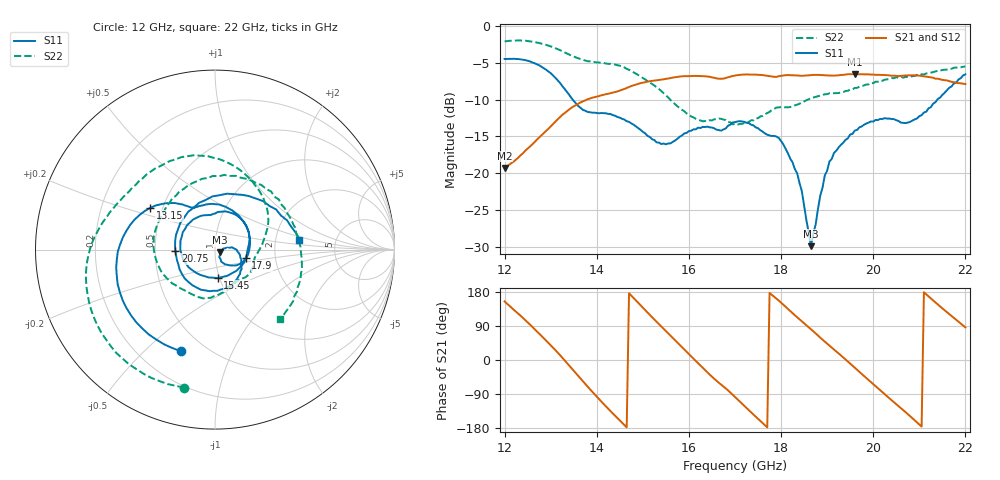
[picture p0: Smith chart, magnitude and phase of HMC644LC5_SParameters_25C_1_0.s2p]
!Analog Devices Inc..
!GaAs MMIC 5-BIT DIGITAL PHASE SHIFTER, 15 -8.5 GHz
!Filename: HMC644LC5_sparm_25C_1_0.s2p
!  :25C = 25degC
!  :_1_ = Sn1
!  :_0  = 0 state (reference)
!Device type:
!2 Port Calibration to sma connectors
!Phase Shifter:  0.000
!	TA = +25deg C, 50 Ohm System, Control Voltage = 0/-3V
!Freq	S11	S11	S21	S21	S12	S12	S22	S22
! GHz	Mag dB	Degrees	Mag dB	Degrees	Mag dB	Degrees	Mag dB	Degrees
# GHZ S DB R 50.0
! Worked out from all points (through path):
!   201 points, 12 GHz to 22 GHz, reference 50 ohm
!   highest |S21| = -6.52 dB at 19.6 GHz (marker M1); lowest = -19.3 dB at 12 GHz (marker M2)
!   lowest |S11| = -29.9 dB at 18.65 GHz (marker M3), VSWR 1.07, Z = 52.9 - j1.58 ohm
!   |S11| at or under -10 dB: 13.48 GHz to 21.39 GHz (7.912 GHz wide, 45.4 % of centre)
!   |S22| runs from -13.4 to -2.0 dB; largest |S21 - S12| = 0.0051
!   S11 on the Smith chart (normalised r, x): 12 GHz: 0.37, -0.65; 13.15 GHz: 0.43, +0.24; 15.45 GHz: 0.98, -0.32; 17.9 GHz: 1.41, -0.13; 20.75 GHz: 0.64, -0.01; 22 GHz: 2.72, +0.36
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12  -4.47 -108.7  -19.30 154.7  -19.26 154.6  -2.06 -102.5
12.55  -4.80 -160.5  -16.38 93.6  -16.39 93.7  -2.08 -140.5
13.15  -7.36 147.1  -12.70 19.9  -12.72 19.9  -3.13 -179.9
13.7  -11.40 119.5  -10.23 -56.2  -10.21 -56.2  -4.59 150.4
14.15  -11.84 97.4  -9.34 -116.2  -9.36 -116.1  -5.01 126.2
14.65  -12.93 49.6  -8.41 -177.7  -8.41 -177.5  -5.81 91.2
15.35  -15.84 -64.7  -7.32 94.5  -7.30 94.6  -8.56 39.7
15.45  -15.97 -84.2  -7.24 82.5  -7.22 82.6  -9.12 32.2
16.15  -14.03 158.3  -6.77 -2.6  -6.77 -2.5  -12.61 -5.8
16.55  -13.90 109.0  -7.03 -49.6  -7.01 -49.5  -12.67 -24.3
17  -13.06 69.7  -6.72 -97.4  -6.70 -97.3  -13.31 -52.5
17.5  -13.89 17.0  -6.62 -155.3  -6.59 -155.2  -12.52 -76.0
17.9  -15.03 -15.2  -6.90 161.8  -6.87 161.9  -11.07 -103.3
18.35  -20.02 -55.7  -6.71 112.5  -6.73 112.5  -10.67 -134.8
18.65  -29.93 -27.9  -6.67 81.0  -6.66 80.9  -9.80 -158.2
18.7  -28.19 -8.5  -6.63 75.7  -6.64 75.5  -9.72 -162.2
19.05  -18.41 -0.1  -6.72 37.8  -6.70 37.8  -9.13 167.2
19.6  -14.21 -44.3  -6.52 -20.6  -6.55 -20.6  -8.41 121.4
20.35  -12.57 -122.3  -6.70 -101.2  -6.69 -100.9  -7.19 57.3
20.75  -13.12 -177.9  -6.70 -142.7  -6.69 -142.6  -6.94 28.1
21.4  -9.92 77.5  -7.15 146.6  -7.12 146.7  -6.08 -12.6
22  -6.56 6.4  -7.88 86.1  -7.92 86.0  -5.49 -46.9
